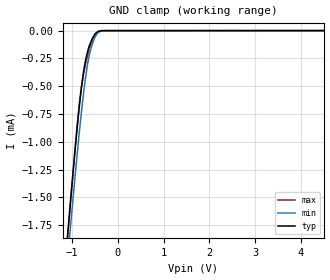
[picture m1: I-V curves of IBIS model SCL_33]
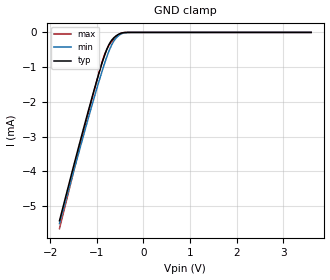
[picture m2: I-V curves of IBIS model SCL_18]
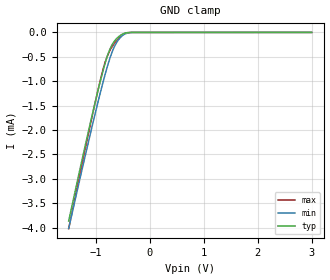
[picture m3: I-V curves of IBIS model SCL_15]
|Texas Instruments Incorporated
|(TMP112)High-Accuracy, Low-Power, Digital Temperature Sensor
|   With SMBus/Two-Wire Serial Interface in SOT563
|(TMP102)Low Power Digital Temperature Sensor
|   With SMBus/Two-Wire Serial Interface in SOT563
| Marketing part#   Digital Voltage Range   Package-type   #pins
|TMP112AIDRLR   1.4 to 3.6   SOT   6
|TMP112AIDRLT   1.4 to 3.6   SOT   6
|TMP102AIDRLR   1.4 to 3.6   SOT   6
|TMP102AIDRLRG4   1.4 to 3.6   SOT   6
|TMP102AIDRLT   1.4 to 3.6   SOT   6
|TMP102AIDRLTG4   1.4 to 3.6   SOT   6
[IBIS Ver]   4.0
[File name]   tmp102_12.ibs
|   SIMDE V2.0 201002
[File Rev]   1.0
[Date]   09/16/2010
[Source]   Texas Instruments Incorporated.
   Analog-eLab, HPA
   12500 TI Blvd
   Dallas, TX -75243
   For Support e-mail: elab_ibis@list.ti.com
[Notes]   Revision History:
   1.0: 09/16/2010
   - Initial version of the model
   - Initial Model generated from simulations in TISPICED
   - Model names with a trailing _33 contains the model for
   3.3V (3.0V and 3.6V).
   - Model names with trailing _18 contains
   the model for 1.8V (1.62V and 1.98V) operation.
   - Model names with trailing _15 contains the model for 1.5V
   (1.4V and 1.6V)operation.
   - Model not matched to measurements
   - C_comp although listed in numerical order of value are
   obtained from varying PVT conditions. For PVT conditions
   for each specific value refer the buffer description under
   respective [Model]. IBIS model user is responsible for using
   appropriate C_comp to simulate for Signal Integrity.
[Disclaimer]
 This product is designed as an aid for customers of Texas Instruments.
 No warranties, either expressed or implied, with respect to this third
 party software (if any) or with respect to its fitness for any
 particular purpose is claimed by Texas Instruments or the author. The
 software (if any) is provided solely on an "as is" basis. The entire
 risk as to its quality and performance is with the customer
[Copyright] (C) Copyright 2010 Texas Instruments Incorporated.
   All rights reserved.
|   TMP112 and TMP102
[Component]   tmp112drl
[Manufacturer] TI
[Package]   | 6 pin SOT - DRL package
| variable   typ   min   max
R_pkg  2.90200E-02   2.51000E-03   5.55300E-02
L_pkg  8.44385E-01nH 8.08430E-01nH 8.79630E-01nH
C_pkg  1.85643E-01pF 1.04670E-01pF 2.66430E-01pF
[Pin] signal_name  model_name  R_pin  L_pin C_pin
1   SCL   SCL   0.05553  0.80991nH  0.10467pF
2   GND   GND   0.00157  0.56488nH  0.18891pF
3   ALERT  ALERT   0.00251  0.87963nH  0.26643pF
4   ADD0   ADD0   0.05553  0.80843nH  0.10508pF
5   V+   POWER   0.00157  0.56488nH  0.18890pF
6   SDA   SDA   0.00251  0.87957nH  0.26639pF
|   Model Selectors
[Model Selector]  SCL
SCL_33   3.3V digital input
SCL_18   1.8V digital input
SCL_15   1.5V digital input
|NOTES   Model SCL split into two Models SCL_33, SCL_18, and SCL_15
|   to accomodate vast voltage range of 1.4 to 3.6V
|   SCL_33 operates in voltage range of 3.0 - 3.3 - 3.6
|   SCL_18 operates in voltage range of 1.92 - 1.8 - 1.98
|   SCL_15  operates in voltage range of 1.4 -.1.5 - 1.6
|   The max pin frequency for Model SCL is 3.4MHz
|   This is referenced with SCL pin in datasheet
[Model Selector]  ALERT
ALERT_33   3.3V digital open drain
ALERT_18   1.8V digital open drain
ALERT_15   1.5V digital open drain
|NOTES   Model ALERT split into two Models ALERT_33, ALERT_18, and ALERT_15
|   to accomodate vast voltage range of 1.4 to 3.6V
|   ALERT_33 operates in voltage range of 3.0 - 3.3 - 3.6
|   ALERT_18 operates in voltage range of 1.92 - 1.8 - 1.98
|   ALERT_15  operates in voltage range of 1.4 -.1.5 - 1.6
|   The max pin frequency for Model ALERT is 3.4MHz
|   This is referenced with ALERT pin in datasheet
[Model Selector]  ADD0
ADD0_33   3.3V digital input
ADD0_18   1.8V digital input
ADD0_15   1.5V digital input
|NOTES   Model ADD0 split into two Models ADD0_33, ADD0_18, and ADD0_15
|   to accomodate vast voltage range of 1.4 to 3.6V
|   ADD0_33 operates in voltage range of 3.0 - 3.3 - 3.6
|   ADD0_18 operates in voltage range of 1.92 - 1.8 - 1.98
|   ADD0_15  operates in voltage range of 1.4 -.1.5 - 1.6
|   The max pin frequency for Model ADD0 is 3.4MHz
|   This is referenced with ADD0 pin in datasheet
[Model Selector]  SDA
SDA_33  3.3V digital I/O open drain
SDA_18  1.8V digital I/O open drain
SDA_15  1.5V digital I/O open drain
| Models and submodels in the file (12): SCL_33 (Input), SCL_18 (Input), SCL_15 (Input), ALERT_33 (Open_drain), ALERT_18 (Open_drain), ALERT_15 (Open_drain), ADD0_33 (Input), ADD0_18 (Input), ADD0_15 (Input), SDA_33 (I/O_open_drain), SDA_18 (I/O_open_drain), SDA_15 (I/O_open_drain)
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|NOTES   Model SDA split into two Models SDA_33, SDA_18, and SDA_15
|   to accomodate vast voltage range of 1.4 to 3.6V
|   SDA_33 operates in voltage range of 3.0 - 3.3 - 3.6
|   SDA_18 operates in voltage range of 1.92 - 1.8 - 1.98
|   SDA_14  operates in voltage range of 1.4 -.1.5 - 1.6
|   The max pin frequency for Model SDA is 3.4MHz
|   This is referenced with SDA pin in datasheet
|   SCL_33   3.3V digital input Model
[Model] SCL_33
Model_type   Input
| Signals   SCL(1)
Vinl = 0.99
Vinh = 2.31
|   typ   min   max
|   (nom PVT)   (Fast PVT)   (slow PVT)
|Average
C_comp   5.4900360e-13  5.4418680e-13  5.5891860e-13
| Where   nom PVT is  Nominal Process, 3.3V, 27C
|   Fast PVT is Strong Process, 3.6V, -40C
|   Slow PVT is Weak Process, 3.0V, 125C
[Voltage Range]   3.3   3   3.6
[Temperature Range]   27   125   -40
|Ambient Temperature   27   125   -40
[Power Clamp Reference]   3.3   3   3.6
[GND Clamp Reference]   0   0   0
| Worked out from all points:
|   GND clamp passes 1 mA (typ) near -0.91 V on its own axis
[GND Clamp]
|   Voltage   I(typ)   I(min)   I(max)
-3.3V     -13.46mA   -13.1mA    -14.03mA
-1.087V   -1.801mA   -2.021mA   -1.829mA
-1.028V   -1.517mA   -1.747mA   -1.528mA
-938.5mV  -1.107mA   -1.342mA   -1.09mA
-840.7mV  -690.3uA   -922.9uA   -666.5uA
-746.4mV  -369.8uA   -564.8uA   -390.9uA
-669.3mV  -208.8uA   -328.8uA   -249.3uA
-622.2mV  -138.7uA   -224.4uA   -178.2uA
-550.1mV  -68.18uA   -112.6uA   -90.26uA
-431.8mV  -7.715uA   -20.4uA    -8.3uA
-283mV    -626.1nA   -693.1nA   -641.4nA
6.6V      0A         0A         0A
[POWER Clamp]
|   SCR cell for ESD function. Effects occurr above VDD x 2
|   Voltage   I(typ)   I(min)   I(max)
-3.3V     0A         0A         0A
0V        0A         0A         0A
6.6V      0A         0A         0A
|   SCL_18   1.8V digital input Model
[Model] SCL_18
Model_type   Input
| Signals   SCL(1)
Vinl = 0.54
Vinh = 1.26
|   typ   min   max
|   (nom PVT)   (Fast PVT)   (slow PVT)
|Average
C_comp   5.8962220e-13  5.6768840e-13  5.9923480e-13
| Where   nom PVT is  Nominal Process, 1.8V, 27C
|   Fast PVT is Strong Process, 1.98V, -40C
|   Slow PVT is Weak Process, 1.62V, 125C
[Voltage Range]   1.8   1.62   1.98
[Temperature Range]   27   125   -40
|Ambient Temperature   27   125   -40
[Power Clamp Reference]   1.8   1.62   1.98
[GND Clamp Reference]   0   0   0
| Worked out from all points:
|   GND clamp passes 1 mA (typ) near -0.91 V on its own axis
[GND Clamp]
|   Voltage   I(typ)   I(min)   I(max)
-1.8V     -5.422mA   -5.502mA   -5.649mA
-1.266V   -2.675mA   -2.874mA   -2.767mA
-1.017V   -1.467mA   -1.695mA   -1.473mA
-894.6mV  -913.6uA   -1.15mA    -888.4uA
-816.7mV  -598.5uA   -825.2uA   -581.8uA
-750.5mV  -381uA     -577.7uA   -399.9uA
-714.6mV  -291.5uA   -458.9uA   -325.4uA
-648.4mV  -174uA     -278.8uA   -215.6uA
-544mV    -62.85uA   -107.4uA   -83.2uA
-426.2mV  -7.015uA   -17.92uA   -7.862uA
-287.6mV  -738.1nA   -782.2nA   -427nA
3.595V    0A         0A         0A
[POWER Clamp]
|   SCR cell for ESD function. Effects occurr above VDD x 2
|   Voltage   I(typ)   I(min)   I(max)
-1.8V     0A         0A         0A
0V        0A         0A         0A
3.6V      0A         0A         0A
|   SCL_15   1.8V digital input Model
[Model] SCL_15
Model_type   Input
| Signals   SCL(1)
Vinl = 0.45
Vinh = 1.05
|   typ   min   max
|   (nom PVT)   (Fast PVT)   (slow PVT)
|Average
C_comp   5.9438280e-13  5.8018180e-13  6.0447370e-13
| Where   nom PVT is  Nominal Process, 1.5V, 27C
|   Fast PVT is Strong Process, 1.6V, -40C
|   Slow PVT is Weak Process, 1.4V, 125C
[Voltage Range]   1.5   1.4   1.6
[Temperature Range]   27   125   -40
|Ambient Temperature   27   125   -40
[Power Clamp Reference]   1.5   1.4   1.6
[GND Clamp Reference]   0   0   0
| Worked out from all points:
|   GND clamp passes 1 mA (typ) near -0.91 V on its own axis
[GND Clamp]
|   Voltage   I(typ)   I(min)   I(max)
-1.5V     -3.861mA   -4.014mA   -4.019mA
-1.278V   -2.733mA   -2.928mA   -2.827mA
-1.073V   -1.733mA   -1.956mA   -1.758mA
-944.8mV  -1.135mA   -1.37mA    -1.12mA
-859.1mV  -764.8uA   -999uA     -737.7uA
-792.7mV  -514uA     -731.9uA   -507.7uA
-712.5mV  -286.9uA   -452.2uA   -321.2uA
-624.9mV  -142.6uA   -229.6uA   -181.8uA
-516.2mV  -42.52uA   -76.66uA   -56.11uA
-413.8mV  -5.086uA   -14.06uA   -7.981uA
-283.3mV  -720.1nA   -701.7nA   -385nA
2.995V    0A         0A         0A
[POWER Clamp]
|   SCR cell for ESD function. Effects occurr above VDD x 2
|   Voltage   I(typ)   I(min)   I(max)
-1.5V     0A         0A         0A
0V        0A         0A         0A
3V        0A         0A         0A
